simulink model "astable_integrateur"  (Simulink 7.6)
settings: Solver=ode14x  StartTime=0.0  StopTime=0.0001  RelTol=1e-3
StopFcn:
  | close all, clc
  | load astable_int.mat
  | plotyy(x(1,:),x(2,:),x(1,:),x(3,:))
  | title('Générateur de signal carré par astable avec intégrateur')
  | xlabel('temps')
  | grid
libraries: fl_lib x8, nesl_utility x3, elec_lib x2

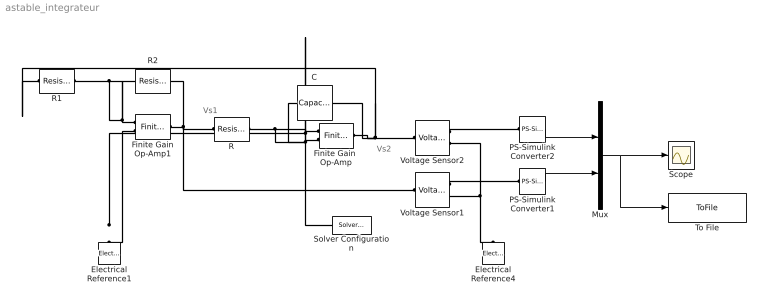
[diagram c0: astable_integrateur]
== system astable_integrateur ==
  note: Vs1
  note: Vs2
  C : fl_lib/Electrical/Electrical Elements/Capacitor  DialogController=NetworkEngine.DynNeDlgSource  SystemSampleTime=-1  c=100 nF  v0=1 V  r=1e-6 Ohm  g=0 1/Ohm  i_Log=off  v_Log=off  vc_Log=off  LocalVarNames=|i|v|vc  LocalVarDescs=|i|v|Internal variable for voltage across capacitor term  LocalVarLogging=[0 0 0]
  Electrical Reference1 : fl_lib/Electrical/Electrical Elements/Electrical Reference  DialogController=NetworkEngine.DynNeDlgSource  SystemSampleTime=-1  i_Log=off  LocalVarNames=|i  LocalVarDescs=|i  LocalVarLogging=[]
  Electrical Reference4 : fl_lib/Electrical/Electrical Elements/Electrical Reference  DialogController=NetworkEngine.DynNeDlgSource  SystemSampleTime=-1  i_Log=off  LocalVarNames=|i  LocalVarDescs=|i  LocalVarLogging=[]
  Finite Gain Op-Amp1 : elec_lib/Integrated Circuits/Finite Gain Op-Amp  DialogController=NetworkEngine.DynNeDlgSource  SystemSampleTime=-1  A=1000  Rin=1e+6 Ohm  Rout=100 Ohm  Vmin=-15 V  Vmax=15 V  LocalVarLogging=[]
  Finite Gain  Op-Amp : elec_lib/Integrated Circuits/Finite Gain Op-Amp  DialogController=NetworkEngine.DynNeDlgSource  SystemSampleTime=-1  A=1000  Rin=1e+6 Ohm  Rout=100 Ohm  Vmin=-15 V  Vmax=15 V  LocalVarLogging=[]
  Mux : Mux  Inputs=2
  PS-Simulink Converter1 : nesl_utility/PS-Simulink Converter  DialogController=NetworkEngine.DynNeUtilDlgSource  SystemSampleTime=-1  PhysicalDomain=network_engine_domain  LeftPortType=input  RightPortType=output  SubClassName=ps_output  Unit=1  AffineConversion=off
  PS-Simulink Converter2 : nesl_utility/PS-Simulink Converter  DialogController=NetworkEngine.DynNeUtilDlgSource  SystemSampleTime=-1  PhysicalDomain=network_engine_domain  LeftPortType=input  RightPortType=output  SubClassName=ps_output  Unit=1  AffineConversion=off
  R : fl_lib/Electrical/Electrical Elements/Resistor  DialogController=NetworkEngine.DynNeDlgSource  SystemSampleTime=-1  R=1 kOhm  i_Log=off  v_Log=off  LocalVarNames=|current|voltage|power  LocalVarDescs=|Resistor current (A)|Voltage across resistor (V)|Power (W)  LocalVarLogging=[0 0 0]
  R1 : fl_lib/Electrical/Electrical Elements/Resistor  DialogController=NetworkEngine.DynNeDlgSource  SystemSampleTime=-1  R=1 kOhm  i_Log=off  v_Log=off  LocalVarNames=|current|voltage|power  LocalVarDescs=|Resistor current (A)|Voltage across resistor (V)|Power (W)  LocalVarLogging=[0 0 0]
  R2 : fl_lib/Electrical/Electrical Elements/Resistor  DialogController=NetworkEngine.DynNeDlgSource  SystemSampleTime=-1  R=47 kOhm  i_Log=off  v_Log=off  LocalVarNames=|current|voltage|power  LocalVarDescs=|Resistor current (A)|Voltage across resistor (V)|Power (W)  LocalVarLogging=[0 0 0]
  Scope : Scope
  Solver Configuration : nesl_utility/Solver Configuration  DialogController=NetworkEngine.DynNeUtilDlgSource  SystemSampleTime=-1  PhysicalDomain=network_engine_domain  LeftPortType=input  RightPortType=generic  SubClassName=solver  Accelerate=off  Profile=off  ResidualTolerance=1e-9  MaxNonlinIter=12  MaxModeIter=2  DoFixedCost=off  UseLocalSampling=off  DoDC=off  LinearAlgebra=Sparse  LocalSolverSampleTime=.001  LocalSolverChoice=NE_BACKWARD_EULER_ADVANCER  UseLocalSolver=off
  To File : ToFile  Filename=astable_int.mat  MatrixName=x
  Voltage Sensor1 : fl_lib/Electrical/Electrical Sensors/Voltage Sensor  DialogController=NetworkEngine.DynNeDlgSource  SystemSampleTime=-1  i1_Log=off  v1_Log=off  LocalVarNames=|i1|v1  LocalVarDescs=|i1|v1  LocalVarLogging=[]
  Voltage Sensor2 : fl_lib/Electrical/Electrical Sensors/Voltage Sensor  DialogController=NetworkEngine.DynNeDlgSource  SystemSampleTime=-1  i1_Log=off  v1_Log=off  LocalVarNames=|i1|v1  LocalVarDescs=|i1|v1  LocalVarLogging=[]
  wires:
  PS-Simulink Converter2/1 -> Mux/1
  PS-Simulink Converter1/1 -> Mux/2
  Mux/1 -> Scope/1, To File/1
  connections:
  Finite Gain  Op-Amp/RConn1 -- C/RConn1 -- R1/LConn1 -- Voltage Sensor2/LConn1
  Finite Gain Op-Amp1/RConn1 -- R2/RConn1 -- Voltage Sensor1/LConn1 -- R/LConn1
  Finite Gain Op-Amp1/LConn2 -- Solver Configuration/RConn1 -- Finite Gain  Op-Amp/LConn1 -- Electrical Reference1/LConn1
  Finite Gain  Op-Amp/LConn2 -- C/LConn1 -- R/RConn1
  Voltage Sensor2/RConn2 -- Electrical Reference4/LConn1 -- Voltage Sensor1/RConn2
  Voltage Sensor2/RConn1 -- PS-Simulink Converter2/LConn1
  Voltage Sensor1/RConn1 -- PS-Simulink Converter1/LConn1
  Finite Gain Op-Amp1/LConn1 -- R2/LConn1 -- R1/RConn1
